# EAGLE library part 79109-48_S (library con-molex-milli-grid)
RECEPTACAL
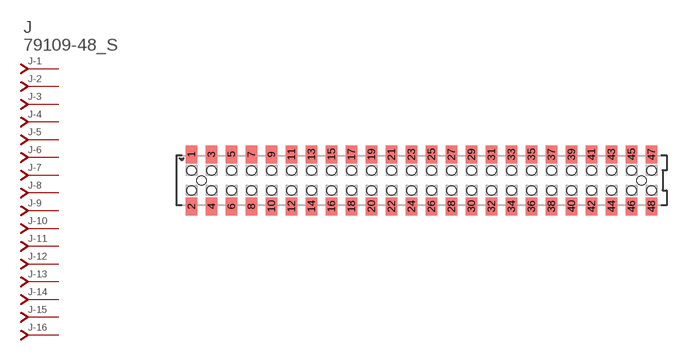
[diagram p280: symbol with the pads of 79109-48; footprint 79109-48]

Designator prefix J; gates -1=J-NV -2=J-N -3=J-N -4=J-N -5=J-N -6=J-N -7=J-N -8=J-N -9=J-N -10=J-N -11=J-N -12=J-N -13=J-N -14=J-N -15=J-N -16=J-N -17=J-N -18=J-N -19=J-N -20=J-N -21=J-N -22=J-N -23=J-N -24=J-N -25=J-N -26=J-N -27=J-N -28=J-N -29=J-N -30=J-N -31=J-N -32=J-N -33=J-N -34=J-N -35=J-N -36=J-N -37=J-N -38=J-N -39=J-N -40=J-N -41=J-N -42=J-N -43=J-N -44=J-N -45=J-N -46=J-N -47=J-N -48=J-N

## 79109-48_S  [79109-48]
1  -1:J  pas
2  -2:J  pas
3  -3:J  pas
4  -4:J  pas
5  -5:J  pas
6  -6:J  pas
7  -7:J  pas
8  -8:J  pas
9  -9:J  pas
10  -10:J  pas
11  -11:J  pas
12  -12:J  pas
13  -13:J  pas
14  -14:J  pas
15  -15:J  pas
16  -16:J  pas
17  -17:J  pas
18  -18:J  pas
19  -19:J  pas
20  -20:J  pas
21  -21:J  pas
22  -22:J  pas
23  -23:J  pas
24  -24:J  pas
25  -25:J  pas
26  -26:J  pas
27  -27:J  pas
28  -28:J  pas
29  -29:J  pas
30  -30:J  pas
31  -31:J  pas
32  -32:J  pas
33  -33:J  pas
34  -34:J  pas
35  -35:J  pas
36  -36:J  pas
37  -37:J  pas
38  -38:J  pas
39  -39:J  pas
40  -40:J  pas
41  -41:J  pas
42  -42:J  pas
43  -43:J  pas
44  -44:J  pas
45  -45:J  pas
46  -46:J  pas
47  -47:J  pas
48  -48:J  pas

## Footprint 79109-48 (pad centres in mm)
RECEPTACAL SMD Dual Row, Vertical, Pass-Thru
smd 1.12 x 1.83: 1 -23,2.6; 2 -23,-2.6; 3 -21,2.6; 4 -21,-2.6; 5 -19,2.6; 6 -19,-2.6; 7 -17,2.6; 8 -17,-2.6; 9 -15,2.6; 10 -15,-2.6; 11 -13,2.6; 12 -13,-2.6; 13 -11,2.6; 14 -11,-2.6; 15 -9,2.6; 16 -9,-2.6; 17 -7,2.6; 18 -7,-2.6; 19 -5,2.6; 20 -5,-2.6; 21 -3,2.6; 22 -3,-2.6; 23 -1,2.6; 24 -1,-2.6; 25 1,2.6; 26 1,-2.6; 27 3,2.6; 28 3,-2.6; 29 5,2.6; 30 5,-2.6; 31 7,2.6; 32 7,-2.6; 33 9,2.6; 34 9,-2.6; 35 11,2.6; 36 11,-2.6; 37 13,2.6; 38 13,-2.6; 39 15,2.6; 40 15,-2.6; 41 17,2.6; 42 17,-2.6; 43 19,2.6; 44 19,-2.6; 45 21,2.6; 46 21,-2.6; 47 23,2.6; 48 23,-2.6
hole 0.914 at -22,0
hole 0.914 at -23,1
hole 0.914 at -23,-1
hole 0.914 at -21,-1
hole 0.914 at -21,1
hole 0.914 at -19,-1
hole 0.914 at -19,1
hole 0.914 at -17,1
hole 0.914 at -17,-1
hole 0.914 at -15,1
hole 0.914 at -15,-1
hole 0.914 at -13,1
hole 0.914 at -13,-1
hole 0.914 at -11,1
hole 0.914 at -11,-1
hole 0.914 at -9,-1
hole 0.914 at -9,1
hole 0.914 at -7,1
hole 0.914 at -7,-1
hole 0.914 at -5,1
hole 0.914 at -5,-1
hole 0.914 at -3,1
hole 0.914 at -3,-1
hole 0.914 at -1,-1
hole 0.914 at -1,1
hole 0.914 at 1,1
hole 0.914 at 3,1
hole 0.914 at 5,1
hole 0.914 at 1,-1
hole 0.914 at 3,-1
hole 0.914 at 5,-1
hole 0.914 at 7,-1
hole 0.914 at 9,-1
hole 0.914 at 11,-1
hole 0.914 at 13,-1
hole 0.914 at 15,-1
hole 0.914 at 7,1
hole 0.914 at 9,1
hole 0.914 at 11,1
hole 0.914 at 13,1
hole 0.914 at 15,1
hole 0.914 at 17,-1
hole 0.914 at 19,-1
hole 0.914 at 17,1
hole 0.914 at 19,1
hole 0.914 at 21,1
hole 0.914 at 23,1
hole 0.914 at 21,-1
hole 0.914 at 23,-1
hole 0.914 at 22,0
